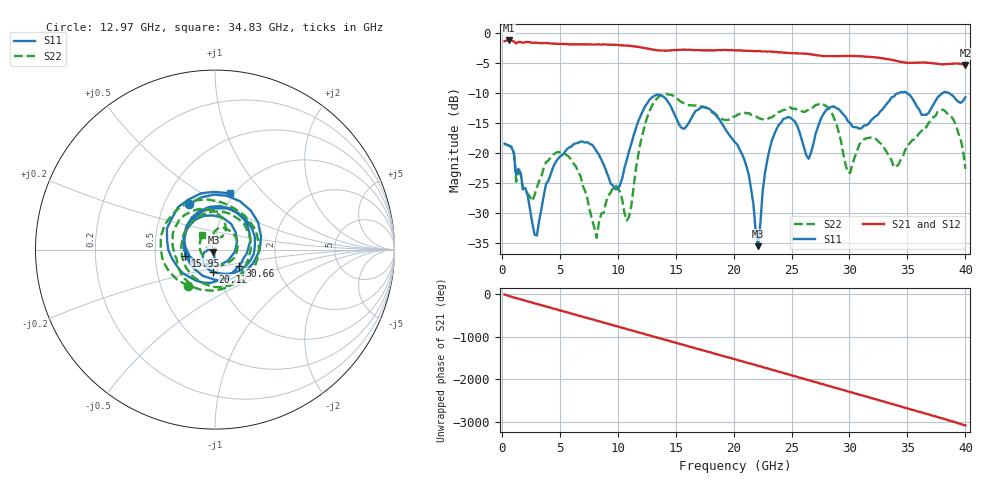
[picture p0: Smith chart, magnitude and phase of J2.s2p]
!Agilent Technologies,E8364B,MY43040528,A.07.50.67
!Agilent E8364B: A.07.50.67
!Date: Thursday, May 22, 2025 22:49:29
!Correction: S11(Full 2 Port(1,2))
!S21(Full 2 Port(1,2))
!S12(Full 2 Port(1,2))
!S22(Full 2 Port(1,2))
!S2P File: Measurements: S11, S21, S12, S22:
# Hz S  dB  R 50
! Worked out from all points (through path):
!   201 points, 250 MHz to 40 GHz, reference 50 ohm
!   highest |S21| = -1.20 dB at 647.5 MHz (marker M1); lowest = -5.4 dB at 40 GHz (marker M2)
!   group delay of S21, straight-line fit = 214 ps
!   lowest |S11| = -35.5 dB at 22.11 GHz (marker M3), VSWR 1.03, Z = 49.1 - j1.4 ohm
!   |S11| at or under -10 dB: start of sweep to 34.26 GHz; 34.96 GHz to 38.01 GHz (3.055 GHz wide, 8.37 % of centre); 38.61 GHz to end of sweep
!   |S22| runs from -34.1 to -10.1 dB; largest |S21 - S12| = 0.0064
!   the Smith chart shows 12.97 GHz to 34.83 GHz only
!   S11 on the Smith chart (normalised r, x): 12.97 GHz: 0.67, +0.37; 15.95 GHz: 0.72, -0.05; 20.12 GHz: 0.95, -0.24; 30.66 GHz: 1.29, -0.24; 34.83 GHz: 0.95, +0.67
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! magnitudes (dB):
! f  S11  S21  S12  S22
! 250 MHz  -18.4  -1.3  -1.3  -18.5
! 647.5 MHz  -18.8  -1.2  -1.2  -18.8
! 3.033 GHz  -33.8  -1.6  -1.6  -25.7
! 4.622 GHz  -21.6  -1.7  -1.7  -20.0
! 7.008 GHz  -18.1  -1.9  -1.8  -25.6
! 8.2 GHz  -19.7  -1.9  -1.9  -34.1
! 9.79 GHz  -26.0  -1.9  -2.0  -25.3
! 10.78 GHz  -21.2  -2.1  -2.1  -31.3
! 12.97 GHz  -10.7  -2.7  -2.7  -12.1
! 13.57 GHz  -10.3  -2.9  -2.9  -10.5
! 15.95 GHz  -15.5  -2.8  -2.7  -11.9
! 20.12 GHz  -18.2  -2.9  -2.9  -13.9
! 21.32 GHz  -23.6  -2.9  -3.0  -13.3
! 22.11 GHz  -35.5  -3.0  -3.0  -14.1
! 23.7 GHz  -16.0  -3.1  -3.2  -13.4
! 26.88 GHz  -18.5  -3.6  -3.6  -12.3
! 29.86 GHz  -14.7  -3.8  -3.8  -23.2
! 30.66 GHz  -15.7  -3.8  -3.8  -19.6
! 33.44 GHz  -11.3  -4.4  -4.4  -20.5
! 34.83 GHz  -9.8  -4.9  -4.9  -19.4
! 38.01 GHz  -10.0  -5.2  -5.2  -12.7
! 40 GHz  -10.7  -5.4  -5.3  -22.6
